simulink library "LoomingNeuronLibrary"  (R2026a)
settings: Solver=VariableStepAuto
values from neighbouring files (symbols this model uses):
  K_photoD = 1.1536    [FFIModelParams_16_02_2021.m]
  K_photoP = 6.8945    [FFIModelParams_16_02_2021.m]
undefined symbols (not defined in the file or in its folder): alpha_1, alpha_2, DiscIntNeverNeededParam, randi, retinaStencil, tau
libraries: simulink x4, $bdroot x2

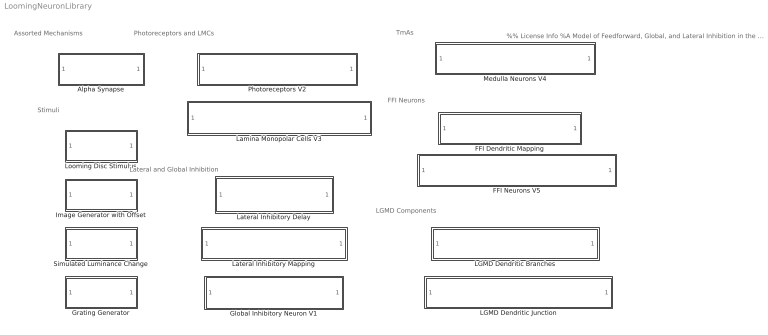
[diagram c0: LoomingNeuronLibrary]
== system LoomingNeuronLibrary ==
  note: TmAs
  note: FFI Neurons
  note: LGMD Components
  note: Lateral and Global Inhibition
  note: Photoreceptors and LMCs
  note: Stimuli
  note: Assorted Mechanisms
  note: %% License Info %A Model of Feedforward, Global, and Lateral Inhibition in the Locust Visual System. %This model examines the architecture and function of inhibitory mechanisms in the %visual system of locusts, namely those involved in the processing of inputs to a %key looming-sensitive neuron, the lobula giant movement detector (LGMD). %Copyright (c) 2026, Erik Olson, Travis Wiens, and Jack Gray %CITATION: %When using the model code for scientific publications, cite the following work: %Olson EGN, Wiens TK, Gray JR. A model of feedforward, global, and lateral inhibition %in the locust visual system predicts responses to looming stimuli. Biol Cybern. 2021 %Jun;115(3):245-265. doi: 10.1007/s00422-021-00876-8. Epub 2021 May 16. PMID: 33997912. %This program is free software: you can redistribute it and/or modify %it under the terms of the GNU General Public License as published by %the Free Software Foundation, either version 3 of the License, or %(at your option) any later version. %This program is distributed in the hope that it will be useful, %but WITHOUT ANY WARRANTY; without even the implied warranty of %MERCHANTABILITY or FITNESS FOR A PARTICULAR PURPOSE. See the %GNU General Public License for more details. %You should have received a copy of the GNU General Public License %along with this program. If not, see <https://www.gnu.org/licenses/>. %Contact: erik.olson@usask.ca
  Alpha Synapse : Subsystem  mask(Synaptic conductance function){tau=tau}
      mask prompts: tau "Synaptic time constant [s]"
      mask help: This block describes an alpha synapse with a single time constant, tau [s] governing peak time and decay. The output is normalized to a peak value of 1.
  FFI Dendritic Mapping : Subsystem  mask(FFI Neuron Dendrites){r_f=0, r_s=0, pop_FFI=0}
      mask prompts: r_f "Receptive field radius"; r_s "Receptive field spacing"; pop_FFI "FFI neuron population size"
      mask help: This block groups LMC outputs into receptive fields corresponding to each FFI neuron. These receptive fields are distributed in a manner mirroring the hexagonal arrangement of the retinotopic units, but with wider spacing of multiple retinotopic units (specified in the parameters). These receptive fields are similarly hexagonal, with sizes specified as a radius in retinotopic units. Inputs: Inputs: TmA Outputs = nondimensionalized alpha synapse outputs from TmAs. Outputs: Inputs to FFI Neurons = vector with elements corresponding to the population size of FFI neurons. Each value represents non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
  FFI Neurons V5 : Subsystem  mask(Feedforward Inhibitory Neurons){K_in=0, g_m=0, c_m=0.1, E_rev=0, E_rest=0, V_t=0, Delta_t=0.001, V_fire=0, tau=0.003, g_FFI_adap=0, tau_FFI_adap=0, E_adap=0, g_noise=0, noise_T=0, pop=0}
      mask prompts: K_in "Input conductance gain"; g_m "Membrane conductance [S/m^2]"; c_m "Membrane capacitance [F/m^2]"; E_rev "Input reversal potential [V]"; E_rest "Membrane resting potential [V]"; V_t "Sodium channel threshold [V]"; Delta_t "Spike initiation sharpness [V]"; V_fire "Firing voltage [V]"; tau "Synaptic decay constant [s]"; g_FFI_adap "Adaptation increment [S/m^2]"; tau_FFI_adap "Adaptation decay constant [s]"; E_adap "Adaptation reversal potential [V]"; g_noise "Noise amplitude [S/m^2]"; noise_T "Noise correlation time [s]"; pop "FFI neuron population size"
      mask help: Models a population of medullary neurons in the locust responsible for feedforward inhibition to the LGMD. Inputs from the lamina should be routed through the corresponding block "FFI Dendritic Mapping" before being supplied to this component. The neurons use an Exponential-Integrate-and-Fire (EIF) Model, incorporating an exponential activation function for sodium currents. The threshold voltage governing these channels is specified separately from the voltage used in spike determination. The neurons also incorporate adaptation currents, albeit without voltage coupling. Noise is also present i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
  Global Inhibitory Neuron V1 : Subsystem  mask(Nonspiking Global Inhibitory Neuron){K_in=0}
      mask prompts: K_in "Input gain [1/V]"
      mask help: This block represents a network of gap junction-connected, nonspiking neurons, receiving excitatory inputs from individual lamina units and generating an inhibitory signal applied across the medulla. The output approaches a limit asymptotically as the input strength increases, simulating the membrane voltage approaching the reversal potential of the input channels. Inputs: Summed LMC Activity = LMC membrane voltages, summed across the entire retina [V] Outputs: Global Inhibitory Signal = nondimensional signal ranging from 0 asymptotically toward a maximum possible value of 1, representing glob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
  Grating Generator : Subsystem  mask{radius=49, theta_max=pi, gratingPeriod=0.2}
      mask prompts: radius "Radius of the eye, in ommatidia"; theta_max "Maximum visual subtense of the eye [rad]"; gratingPeriod "Grating period [rad]"
      mask help: Generates a patch of sinusoidal black and white grating in the center of the visual field, which can move as the "position" input changes. The image background is white. Values regarding the size of the eye in terms of ommatidia and subtense angle are specified in the parameters field. "Grating period" describes the spacing between the dark stripes on the grating. Note that the grating region is rounded up in size to fully occupy any ommatidia near its edge. Inputs: theta = the visual subtense angle of the grating [radians] position = the angular position of the grating [rad]. Increasing or de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
  Image Generator with Offset : Subsystem  mask{radius=49, theta_max=pi, h_offset=0, v_offset=0}
      mask prompts: radius "Radius, in ommatidia"; theta_max "Maximum visual subtense [rad]"; h_offset "Axis 1 offset of image, in ommatidia"; v_offset "Axis 2 offset of image"
      mask help: Generates an array of luminance inputs to a simulated compound eye. These inputs correspond to the image of an approaching black disc-shaped object on a white background. The data is stored in a portion of a square array with the corners removed, corresponding to a hexagonal array of hexagonal ommatidia. The center of the image can be offset from the center of the eye along two axes by integer numbers of ommatidia. Due to the hexagonal nature of the ommatidial arrangement, these two axes are 60 degrees apart. Inputs: theta = the visual subtense angle of the object [radians] Outputs: image = a 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
  LGMD Dendritic Branches : Subsystem  mask(LGMD Dendritic Field A Branches){K_in=0, A_m=5e-6, G_m=0, G_b_j=0, C_m=1e-5, E_rev=0, E_rest=-0.07}
      mask prompts: K_in "Input conductance gain [S]"; A_m "Membrane area [m^2]"; G_m "Membrane conductance [S/m^2]"; G_b_j "Dendrite-soma conductance [S]"; C_m "Membrane capacitance [F/m^2]"; E_rev "Input reversal potential [V]"; E_rest "Resting potential [V]"
      mask help: A simulation of the branches of LGMD dendritic field A for a compartmental model. Inputs: TmA Outputs = nondimensionalized alpha synapse outputs from TmAs; these must first be correctly mapped into a vector corresponding in size to the number of dendritic branches. Dendritic Junction Membrane Voltage = membrane potential [V] of the attached dendritic junction compartment, used to determine intercompartmental currents. Outputs: Dendrite Voltages = vector of membrane potentials [V] of the modelled dendrites, used for monitoring purposes. Output Current = total output current from the dendrititic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
  LGMD Dendritic Junction : Subsystem  mask(LGMD Dendritic Field A Branches){A_m=5e-9, G_j_c=0, G_m=1.1, C_m=0.015, E_rest=0}
      mask prompts: A_m "Membrane Area [m^2]"; G_j_c "Junction-calcium conductance [S]"; G_m "Membrane conductance [S/m^2]"; C_m "Membrane capacitance [F/m^2]"; E_rest "Resting potential [mV]"
      mask help: A simulation of the proximal portion of LGMD dendritic field A. Inputs: Calcium Compartment Membrane Voltage = membrane potential [V] of the attached calcium compartment, used to determine intercompartmental currents. Dendritic Currents = total input current from the dendrititic branches to the dendritic junction compartment [A]. Outputs: Output Currents = total output current from the dendrititic junction to the calcium compartment [A]. Membrane Voltage = membrane potential [V] of the dendritic junction, used for monitoring purposes.
  Lamina Monopolar Cells V3 : Subsystem  mask(Locust Lamina Monopolar Cells){K_LMC=0, gamma_1=0}
      mask prompts: K_LMC "Gain [1/s]"; gamma_1 "Pole [1/s]"
      mask help: A representation of locust lamina monopolar cells. Uses a first-order transfer function with a single zero to approximate the response of lamina monopolar cell membrane voltage to photoreceptor membrane voltage. The response modelled is purely transient. Inputs: Photoreceptor Membrane Voltages = membrane potentials [V] of the photoreceptor corresponding to the modelled LMC, or an array thereof Outputs: LMC Membrane Voltages = membrane potentials [V] of corresponding dimensionality to the luminance inputs (either single or an array).
  Lateral Inhibitory Delay : Subsystem  mask(Lateral Inhibitory Delay){tau=1}
      mask prompts: tau "Time constant [s]"
      mask help: A first order low-pass filter, used to delay and temporally broaden LMC excitatory signals for use as lateral inhibition. LMC Activity = membrane potentials [V] of modelled LMCs, in array format Outputs: Lateral Inhibitory Signals = delayed and broadened LMC outputs [V], prior to mapping to adjacent retinotopic units.
  Lateral Inhibitory Mapping : Subsystem  mask(Lamina Output Mapping){stencil=0}
      mask prompts: stencil "Convolution kernel"
      mask help: This block maps signals from adjacent lamina cells to medullary neurons by using a supplied stencil to perform a 2D convolution. Inputs: Lamina Outputs = an array of LMC membrane potentials delayed via low-pass filter [V] Outputs: Lateral Inhibitory Signals = an array of inputs to the TmAs, corresponding to outputs of retinotopically adjacent LMCs, with radius and weightings determined by the kernel used for convolution
  Looming Disc Stimulus : Subsystem  mask(Looming Disc Stimulus){l=.07, v=3, d_0=0}
      mask prompts: l "stimulus half-height [m]"; v "stimulus approach velocity [m/s]"; d_0 "starting distance [m]"
      mask help: To be used in modelling visual parameters of a looming disc-shaped object, based on its half-height, approach velocity, and starting distance. Outputs include: theta = the visual subtense angle [rad] t_collision = simulation time normalized to the time of collision [s], such that negative values represent time pre-collision
  Medulla Neurons V4 : Subsystem  mask(Trans-medullary Afferents){K_in_ex=0, K_in_lateral=0, K_in_global=0, g_m=0, c_m=0.01, E_rev_ex=0, E_rev_inh=0, E_rest=0, V_t=0, Delta_t=0.001, V_fire=0, tau=0.0003, g_med_adap_inc=0, tau_med_adap=0.1, E_rev_adap=0, g_noise=0, noise_T=0.01, radius=1}
      mask prompts: K_in_ex "Excitatory conductance gain [S/(m^2*V)]"; K_in_lateral "Lateral inhibition conductance gain [S/(m^2*V)]"; K_in_global "Global inhibition conductance gain [S/(m^2)]"; g_m "Membrane conductance [S/m^2]"; c_m "Membrane capacitance [F/m^2]"; E_rev_ex "Excitatory reversal potential [V]"; E_rev_inh "Inhibitory reversal potential [V]"; E_rest "Membrane resting potential [V]"; V_t "Spike initiation threshold [V]"; Delta_t "Spike initiation sharpness [V]"; V_fire "Firing voltage [V]"; tau "Synaptic decay constant [s]"; g_med_adap_inc "Adaptation conductance increment [S/m^2]"; tau_med_adap "Adaptation time constant [s]"; E_rev_adap "Adaptation reversal potential [V]"; g_noise "Noise amplitude [S/m^2]"; noise_T "Noise correlation time [s]"; radius "Radius, in ommatidia"
      mask help: These neurons are meant to receive excitatory inputs from a retinotopically correspondent LMC, along with lateral inhibition based on adjacent LMC behaviour and global inhibition based on summed LMC behavior. They use an Exponential-Integrate-and-Fire (EIF) Model, incorporating an exponential activation function for spike initiation representing the function of voltage-gated sodium channels. The threshold voltage governing these channels is specified separately from the voltage used in spike determination. An adaptation current is also implemented; this does not include a voltage coupling term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
  Photoreceptors V2 : Subsystem  mask(Locust Photoreceptors){K_photoD=K_photoD, K_photoP=K_photoP, alpha_1=alpha_1, alpha_2=alpha_2}
      mask prompts: K_photoD "Derivative coefficient [V/s]"; K_photoP "Proportional coefficient [V/s^2]"; alpha_1 "First pole [1/s]"; alpha_2 "Second pole [1/s]"
      mask help: A representation of locust photoreceptors. Uses a 2nd-order transfer function with a single zero to model the response of membrane voltage to luminance, incorporating a transient overshoot and a steady-state component. Inputs: Luminance Values = either a single luminance value ranging from 1 (white) to 0 (black) representing visual input from the corresponding ommatidium, or an array thereof,. Outputs: Photoreceptor Membrane Voltages = membrane voltage of photoreceptors [V], of corresponding dimensionality to the luminance inputs (either single or an array).
  Simulated Luminance Change : Subsystem  mask(Simulated Luminance Change){duration=1, start=0}
      mask prompts: duration "Duration [s]"; start "Start time [s]"
      mask help: Simulates the luminance change from dark to light to over a single ommatidium due to an edge moving at constant speed. Used to implement single-facet stimuli . The luminance corresponds to the potion of a circular region covered by a straight line passing across it at constant speed. Outputs: luminance = a luminance value transition from 1 (white) to 0 (black), starting at the specified time and ending after the specified duration.

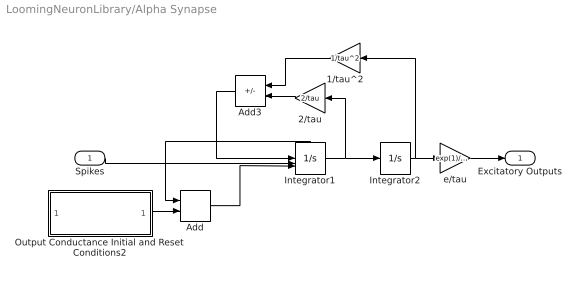
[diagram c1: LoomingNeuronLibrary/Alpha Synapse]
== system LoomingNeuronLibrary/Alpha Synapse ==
  Spikes : Inport
  1/tau^2 : Gain  Gain=1/tau^2
  2/tau : Gain  Gain=2/tau
  Add : Sum
  Add3 : Sum  Inputs=--
  Integrator1 : Integrator  ExternalReset=rising  InitialConditionSource=external  ShowStatePort=on
  Integrator2 : Integrator
  Output Conductance Initial and Reset Conditions2 : Subsystem
  e/tau : Gain  Gain=exp(1)/tau
  Excitatory Outputs : Outport  VectorParamsAs1DForOutWhenUnconnected=off
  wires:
  Add3/1 -> Integrator1/1
  Integrator2/1 -> 1/tau^2/1, e/tau/1
  e/tau/1 -> Excitatory Outputs/1
  Output Conductance Initial and Reset Conditions2/1(Reset Value) -> Add/2
  1/tau^2/1 -> Add3/1
  Add/1 -> Integrator1/3
  Integrator1/1 -> 2/tau/1, Integrator2/1
  Integrator1/State -> Add/1
  Spikes/1 -> Integrator1/2
  2/tau/1 -> Add3/2

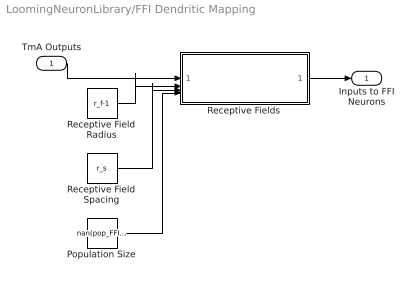
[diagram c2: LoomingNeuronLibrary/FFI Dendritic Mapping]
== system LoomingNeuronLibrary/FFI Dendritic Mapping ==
  TmA Outputs : Inport
  Population Size : Constant  Value=nan(pop_FFI,1)
  Receptive Field Radius : Constant  Value=r_f-1
  Receptive Field Spacing : Constant  Value=r_s
  Receptive Fields : MATLAB Function  TreatAsAtomicUnit=on
  Inputs to FFI Neurons : Outport  VectorParamsAs1DForOutWhenUnconnected=off
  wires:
  Population Size/1 -> Receptive Fields/4(output_array)
  Receptive Field Spacing/1 -> Receptive Fields/3(r_s)
  TmA Outputs/1 -> Receptive Fields/1(LMCs)
  Receptive Field Radius/1 -> Receptive Fields/2(r_f)
  Receptive Fields/1(y) -> Inputs to FFI Neurons/1

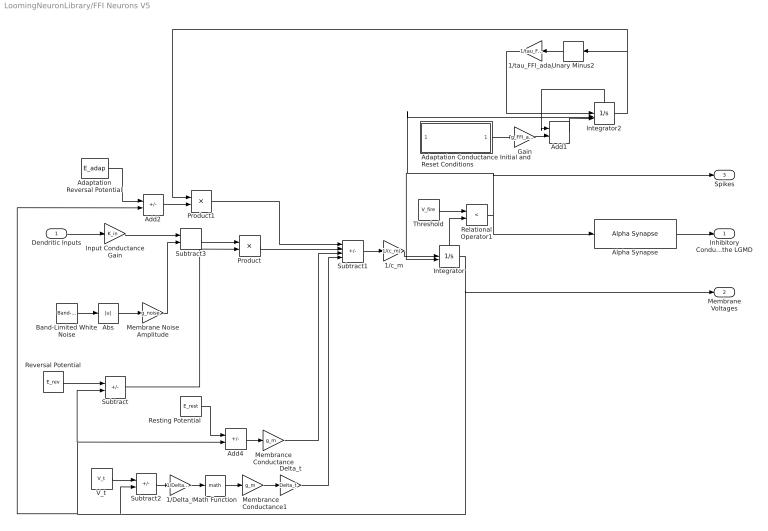
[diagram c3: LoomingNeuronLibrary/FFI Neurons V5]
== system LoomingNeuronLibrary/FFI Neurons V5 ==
  Dendritic Inputs : Inport
  1/Delta_t : Gain  Gain=1/Delta_t
  1/c_m : Gain  Gain=1/(c_m)
  1/tau_FFI_adap : Gain  Gain=1/tau_FFI_adap
  Abs : Abs
  Adaptation Reversal Potential : Constant  Value=E_adap
  Adaptation Conductance Initial and Reset Conditions : Subsystem
  Add1 : Sum
  Add2 : Sum  Inputs=-+
  Add4 : Sum  Inputs=-+
  Alpha Synapse : $bdroot/Alpha Synapse  tau=tau
  Band-Limited White Noise : simulink/Sources/Band-Limited White Noise  Cov=[noise_T]  Ts=noise_T  seed=randi(1000000,pop,1)
  Delta_t : Gain  Gain=Delta_t
  Gain : Gain  Gain=g_FFI_adap
  Input Conductance Gain : Gain  Gain=K_in
  Integrator : Integrator  ExternalReset=rising  InitialCondition=E_rest  ShowStatePort=on
  Integrator2 : Integrator  ExternalReset=rising  InitialConditionSource=external  ShowStatePort=on
  Math Function : Math  SignedPower=on
  Membrance Conductance : Gain  Gain=g_m
  Membrance Conductance1 : Gain  Gain=g_m
  Membrane Noise Amplitude : Gain  Gain=g_noise
  Product : Product
  Product1 : Product
  Relational Operator1 : RelationalOperator  Operator=<  OutDataTypeStr=boolean  RndMeth=Simplest
  Resting Potential : Constant  Value=E_rest
  Reversal Potential : Constant  Value=E_rev
  Subtract : Sum  Inputs=+-
  Subtract1 : Sum  Inputs=-+-+
  Subtract2 : Sum  Inputs=-+
  Subtract3 : Sum
  Threshold : Constant  Value=V_fire
  Unary Minus2 : UnaryMinus
  V_t : Constant  Value=V_t
  Inhibitory Conductance Outputs to the LGMD : Outport  VectorParamsAs1DForOutWhenUnconnected=off
  Membrane Voltages : Outport  Port=2  VectorParamsAs1DForOutWhenUnconnected=off
  Spikes : Outport  Port=3  VectorParamsAs1DForOutWhenUnconnected=off
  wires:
  Threshold/1 -> Relational Operator1/1
  Subtract/1 -> Product/2
  Subtract1/1 -> 1/c_m/1
  Resting Potential/1 -> Add4/1
  Dendritic Inputs/1 -> Input Conductance Gain/1
  1/c_m/1 -> Integrator/1
  Integrator/State -> Relational Operator1/2
  Reversal Potential/1 -> Subtract/1
  Add4/1 -> Membrance Conductance/1
  Subtract2/1 -> 1/Delta_t/1
  Delta_t/1 -> Subtract1/4
  Math Function/1 -> Membrance Conductance1/1
  1/Delta_t/1 -> Math Function/1
  Membrance Conductance1/1 -> Delta_t/1
  V_t/1 -> Subtract2/1
  1/tau_FFI_adap/1 -> Integrator2/1
  Integrator2/State -> Add1/1
  Unary Minus2/1 -> 1/tau_FFI_adap/1
  Relational Operator1/1 -> Alpha Synapse/1, Spikes/1, Integrator2/2, Integrator/2
  Add1/1 -> Integrator2/3
  Gain/1 -> Add1/2
  Integrator2/1 -> Unary Minus2/1, Product1/1
  Product1/1 -> Subtract1/1
  Add2/1 -> Product1/2
  Integrator/1 -> Membrane Voltages/1, Subtract2/2, Add4/2, Subtract/2, Add2/2
  Adaptation Reversal Potential/1 -> Add2/1
  Membrance Conductance/1 -> Subtract1/3
  Product/1 -> Subtract1/2
  Band-Limited White Noise/1 -> Abs/1
  Membrane Noise Amplitude/1 -> Subtract3/2
  Abs/1 -> Membrane Noise Amplitude/1
  Subtract3/1 -> Product/1
  Input Conductance Gain/1 -> Subtract3/1
  Adaptation Conductance Initial and Reset Conditions/1(Reset Value) -> Gain/1
  Alpha Synapse/1 -> Inhibitory Conductance Outputs to the LGMD/1

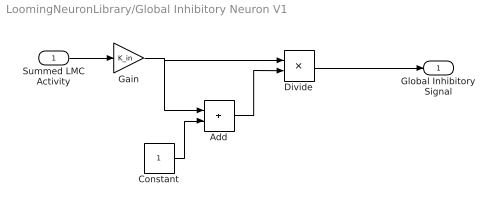
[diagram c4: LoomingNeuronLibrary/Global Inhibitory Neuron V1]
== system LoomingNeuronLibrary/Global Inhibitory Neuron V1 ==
  Summed LMC Activity : Inport
  Add : Sum
  Constant : Constant
  Divide : Product  Inputs=*/
  Gain : Gain  Gain=K_in
  Global Inhibitory Signal : Outport  VectorParamsAs1DForOutWhenUnconnected=off
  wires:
  Divide/1 -> Global Inhibitory Signal/1
  Summed LMC Activity/1 -> Gain/1
  Gain/1 -> Add/1, Divide/1
  Constant/1 -> Add/2
  Add/1 -> Divide/2

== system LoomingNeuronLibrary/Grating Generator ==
  theta : Inport
  position : Inport  Port=2
  Constant : Constant  Value=ones(2*radius-1, 2*radius-1)
  Constant1 : Constant  Value=gratingPeriod
  MATLAB Function : MATLAB Function  TreatAsAtomicUnit=on
  image : Outport  PortDimensions=[2*radius-1 2*radius-1]  VectorParamsAs1DForOutWhenUnconnected=off
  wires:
  theta/1 -> MATLAB Function/1(theta)
  MATLAB Function/1(image) -> image/1
  Constant/1 -> MATLAB Function/4(blank)
  position/1 -> MATLAB Function/2(position)
  Constant1/1 -> MATLAB Function/3(gratingPeriod)

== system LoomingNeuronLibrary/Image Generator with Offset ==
  theta : Inport
  Constant : Constant  Value=ones(2*radius-1, 2*radius-1)
  Constant1 : Constant  Value=h_offset
  Constant2 : Constant  Value=v_offset
  MATLAB Function : MATLAB Function  TreatAsAtomicUnit=on
  image : Outport  PortDimensions=[2*radius-1 2*radius-1]  VectorParamsAs1DForOutWhenUnconnected=off
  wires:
  theta/1 -> MATLAB Function/1(theta)
  MATLAB Function/1(image) -> image/1
  Constant/1 -> MATLAB Function/2(blank)
  Constant1/1 -> MATLAB Function/3(h_offset)
  Constant2/1 -> MATLAB Function/4(v_offset)

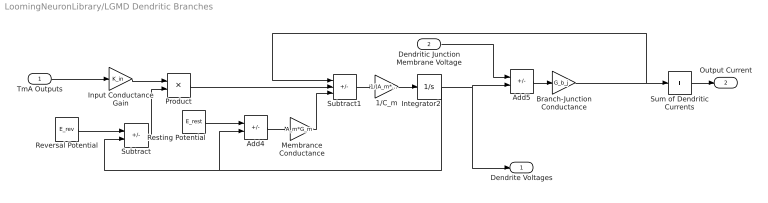
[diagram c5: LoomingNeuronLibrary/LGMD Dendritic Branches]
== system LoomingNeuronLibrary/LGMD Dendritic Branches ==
  TmA Outputs : Inport
  Dendritic Junction Membrane Voltage : Inport  Port=2
  1/C_m : Gain  Gain=1/(A_m*C_m)
  Add4 : Sum  Inputs=-+
  Add5 : Sum  Inputs=-+
  Branch-Junction Conductance : Gain  Gain=G_b_j
  Input Conductance Gain : Gain  Gain=K_in
  Integrator2 : Integrator  InitialCondition=E_rest
  Membrance Conductance : Gain  Gain=A_m*G_m
  Product : Product
  Resting Potential : Constant  Value=E_rest
  Reversal Potential : Constant  Value=E_rev
  Subtract : Sum  Inputs=+-
  Subtract1 : Sum  Inputs=-+-
  Sum of Dendritic Currents : Sum  Inputs=+
  Dendrite Voltages : Outport  VectorParamsAs1DForOutWhenUnconnected=off
  Output Current : Outport  Port=2  VectorParamsAs1DForOutWhenUnconnected=off
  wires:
  1/C_m/1 -> Integrator2/1
  Sum of Dendritic Currents/1 -> Output Current/1
  Integrator2/1 -> Add4/2, Subtract/2, Dendrite Voltages/1, Add5/2
  Subtract/1 -> Product/2
  Reversal Potential/1 -> Subtract/1
  Add4/1 -> Membrance Conductance/1
  Input Conductance Gain/1 -> Product/1
  Subtract1/1 -> 1/C_m/1
  Resting Potential/1 -> Add4/1
  TmA Outputs/1 -> Input Conductance Gain/1
  Dendritic Junction Membrane Voltage/1 -> Add5/1
  Product/1 -> Subtract1/2
  Membrance Conductance/1 -> Subtract1/3
  Add5/1 -> Branch-Junction Conductance/1
  Branch-Junction Conductance/1 -> Subtract1/1, Sum of Dendritic Currents/1

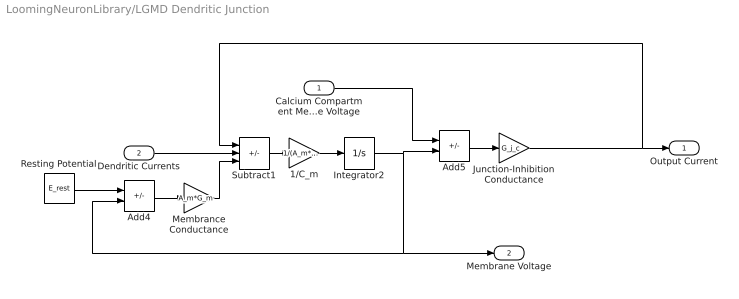
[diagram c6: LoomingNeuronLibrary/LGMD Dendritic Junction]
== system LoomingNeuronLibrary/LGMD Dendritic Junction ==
  Calcium Compartment Membrane Voltage : Inport
  Dendritic Currents : Inport  Port=2
  1/C_m : Gain  Gain=1/(A_m*C_m)
  Add4 : Sum  Inputs=-+
  Add5 : Sum  Inputs=-+
  Integrator2 : Integrator  InitialCondition=E_rest
  Junction-Inhibition Conductance : Gain  Gain=G_j_c
  Membrance Conductance : Gain  Gain=A_m*G_m
  Resting Potential : Constant  Value=E_rest
  Subtract1 : Sum  Inputs=-+-
  Output Current : Outport  VectorParamsAs1DForOutWhenUnconnected=off
  Membrane Voltage : Outport  Port=2  VectorParamsAs1DForOutWhenUnconnected=off
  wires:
  Membrance Conductance/1 -> Subtract1/3
  Add4/1 -> Membrance Conductance/1
  1/C_m/1 -> Integrator2/1
  Dendritic Currents/1 -> Subtract1/2
  Subtract1/1 -> 1/C_m/1
  Resting Potential/1 -> Add4/1
  Add5/1 -> Junction-Inhibition Conductance/1
  Calcium Compartment Membrane Voltage/1 -> Add5/1
  Junction-Inhibition Conductance/1 -> Output Current/1, Subtract1/1
  Integrator2/1 -> Add5/2, Membrane Voltage/1, Add4/2

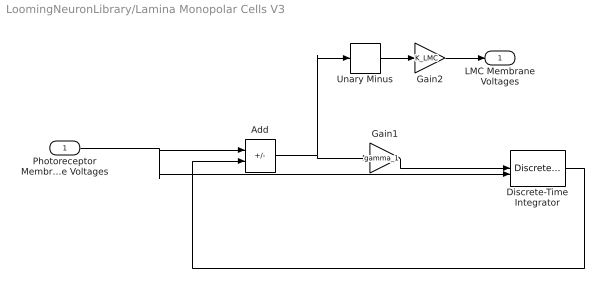
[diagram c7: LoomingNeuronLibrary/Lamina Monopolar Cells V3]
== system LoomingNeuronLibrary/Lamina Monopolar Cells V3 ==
  Photoreceptor Membrane Voltages : Inport
  Add : Sum  Inputs=+-
  Discrete-Time Integrator : DiscreteIntegrator  InitialConditionSource=external  SampleTime=-1  ICPrevOutput=DiscIntNeverNeededParam  ICPrevScaledInput=DiscIntNeverNeededParam
  Gain1 : Gain  Gain=gamma_1
  Gain2 : Gain  Gain=K_LMC
  Unary Minus : UnaryMinus
  LMC Membrane Voltages : Outport  VectorParamsAs1DForOutWhenUnconnected=off
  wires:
  Gain1/1 -> Discrete-Time Integrator/1
  Discrete-Time Integrator/1 -> Add/2
  Photoreceptor Membrane Voltages/1 -> Discrete-Time Integrator/2, Add/1
  Add/1 -> Unary Minus/1, Gain1/1
  Unary Minus/1 -> Gain2/1
  Gain2/1 -> LMC Membrane Voltages/1

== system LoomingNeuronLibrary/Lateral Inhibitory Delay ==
  LMC Activity : Inport
  Add : Sum  Inputs=+-
  Discrete-Time Integrator : DiscreteIntegrator  SampleTime=-1  ICPrevOutput=DiscIntNeverNeededParam  ICPrevScaledInput=DiscIntNeverNeededParam
  Gain : Gain  Gain=1/tau
  Lateral Inhibitory Signals : Outport
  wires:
  Discrete-Time Integrator/1 -> Lateral Inhibitory Signals/1, Add/2
  Add/1 -> Gain/1
  LMC Activity/1 -> Add/1
  Gain/1 -> Discrete-Time Integrator/1

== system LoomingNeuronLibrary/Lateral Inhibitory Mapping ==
  Lamina Outputs : Inport
  Constant : Constant  Value=stencil
  MATLAB Function : MATLAB Function  TreatAsAtomicUnit=on
  Lateral Inhibitory Signals : Outport  VectorParamsAs1DForOutWhenUnconnected=off
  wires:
  Lamina Outputs/1 -> MATLAB Function/1(LMCs)
  MATLAB Function/1(inhibition) -> Lateral Inhibitory Signals/1
  Constant/1 -> MATLAB Function/2(stencil)

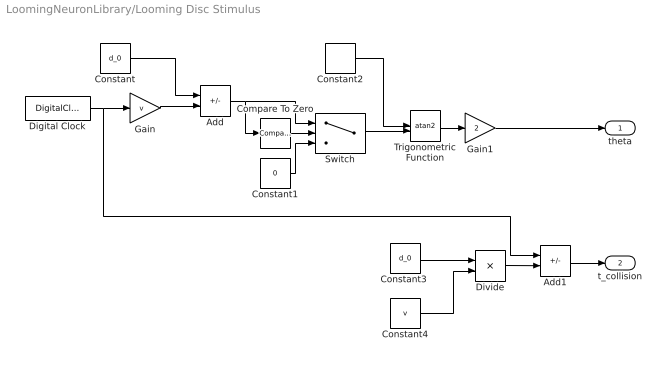
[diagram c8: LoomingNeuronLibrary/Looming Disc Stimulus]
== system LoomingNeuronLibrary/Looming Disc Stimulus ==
  Add : Sum  Inputs=+-
  Add1 : Sum  Inputs=+-
  Compare To Zero : simulink/Logic and Bit Operations/Compare To Zero  relop=>=  OutDataTypeStr=boolean
  Constant : Constant  Value=d_0
  Constant1 : Constant  Value=0
  Constant2 : Constant  Value=l
  "Constant3 " : Constant  Value=d_0
  Constant4 : Constant  Value=v
  Digital Clock : DigitalClock  SampleTime=-1
  Divide : Product  Inputs=*/
  Gain : Gain  Gain=v
  Gain1 : Gain  Gain=2
  Switch : Switch  Criteria=u2 > Threshold
  Trigonometric Function : Trigonometry  Operator=atan2  OutputSignalType=real
  theta : Outport  VectorParamsAs1DForOutWhenUnconnected=off
  t_collision : Outport  Port=2  VectorParamsAs1DForOutWhenUnconnected=off
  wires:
  Constant/1 -> Add/1
  Gain/1 -> Add/2
  Compare To Zero/1 -> Switch/2
  Digital Clock/1 -> Add1/1, Gain/1
  Add/1 -> Compare To Zero/1, Switch/1
  Constant1/1 -> Switch/3
  Trigonometric Function/1 -> Gain1/1
  Switch/1 -> Trigonometric Function/2
  Constant2/1 -> Trigonometric Function/1
  Gain1/1 -> theta/1
  "Constant3 "/1 -> Divide/1
  Constant4/1 -> Divide/2
  Divide/1 -> Add1/2
  Add1/1 -> t_collision/1

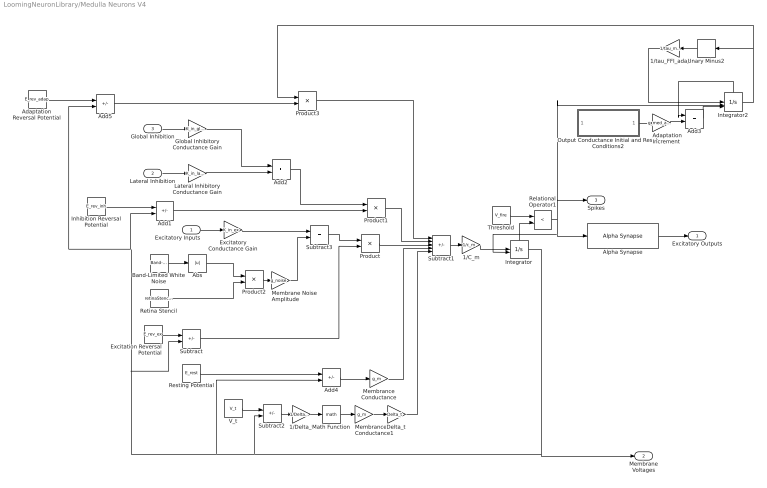
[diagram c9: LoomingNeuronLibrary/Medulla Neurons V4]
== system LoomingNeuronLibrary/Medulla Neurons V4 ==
  Excitatory Inputs : Inport
  Lateral Inhibition : Inport  Port=2
  Global Inhibition : Inport  Port=3
  1/C_m : Gain  Gain=1/c_m
  1/Delta_t : Gain  Gain=1/Delta_t
  1/tau_FFI_adap : Gain  Gain=1/tau_med_adap
  Abs : Abs
  Adaptation Increment : Gain  Gain=g_med_adap_inc
  Adaptation Reversal Potential : Constant  Value=E_rev_adap
  Add1 : Sum  Inputs=-+
  Add2 : Sum
  Add3 : Sum
  Add4 : Sum  Inputs=-+
  Add5 : Sum  Inputs=-+
  Alpha Synapse : $bdroot/Alpha Synapse  tau=tau
  Band-Limited White Noise : simulink/Sources/Band-Limited White Noise  Cov=[noise_T]  Ts=noise_T  seed=randi(1000000,2*radius-1)
  Delta_t : Gain  Gain=Delta_t
  Excitation Reversal Potential : Constant  Value=E_rev_ex
  Excitatory Conductance Gain : Gain  Gain=K_in_ex
  Global Inhibitory Conductance Gain : Gain  Gain=K_in_global
  Inhibition Reversal Potential : Constant  Value=E_rev_inh
  Integrator : Integrator  ExternalReset=rising  InitialCondition=E_rest  ShowStatePort=on
  Integrator2 : Integrator  ExternalReset=rising  InitialConditionSource=external  ShowStatePort=on
  Lateral Inhibitory Conductance Gain : Gain  Gain=K_in_lateral
  Math Function : Math  SignedPower=on
  Membrance Conductance : Gain  Gain=g_m
  Membrance Conductance1 : Gain  Gain=g_m
  Membrane Noise Amplitude : Gain  Gain=g_noise
  Output Conductance Initial and Reset Conditions2 : Subsystem
  Product{,1..3} (4 alike) : Product
  Relational Operator1 : RelationalOperator  Operator=<  OutDataTypeStr=boolean  RndMeth=Simplest
  Resting Potential : Constant  Value=E_rest
  Retina Stencil : Constant  Value=retinaStencil(radius)
  Subtract : Sum  Inputs=+-
  Subtract1 : Sum  Inputs=--+-+
  Subtract2 : Sum  Inputs=-+
  Subtract3 : Sum
  Threshold : Constant  Value=V_fire
  Unary Minus2 : UnaryMinus
  V_t : Constant  Value=V_t
  Excitatory Outputs : Outport  VectorParamsAs1DForOutWhenUnconnected=off
  Membrane Voltages : Outport  Port=2  VectorParamsAs1DForOutWhenUnconnected=off
  Spikes : Outport  Port=3  VectorParamsAs1DForOutWhenUnconnected=off
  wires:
  Global Inhibition/1 -> Global Inhibitory Conductance Gain/1
  Integrator/State -> Relational Operator1/2
  Product/1 -> Subtract1/3
  Excitation Reversal Potential/1 -> Subtract/1
  Resting Potential/1 -> Add4/1
  Product1/1 -> Subtract1/2
  Delta_t/1 -> Subtract1/5
  1/Delta_t/1 -> Math Function/1
  Threshold/1 -> Relational Operator1/1
  Add4/1 -> Membrance Conductance/1
  Subtract2/1 -> 1/Delta_t/1
  Math Function/1 -> Membrance Conductance1/1
  Subtract/1 -> Product/2
  V_t/1 -> Subtract2/1
  Membrance Conductance/1 -> Subtract1/4
  Excitatory Inputs/1 -> Excitatory Conductance Gain/1
  Alpha Synapse/1 -> Excitatory Outputs/1
  Membrance Conductance1/1 -> Delta_t/1
  Subtract1/1 -> 1/C_m/1
  Lateral Inhibition/1 -> Lateral Inhibitory Conductance Gain/1
  Inhibition Reversal Potential/1 -> Add1/1
  1/C_m/1 -> Integrator/1
  Add2/1 -> Product1/1
  Add1/1 -> Product1/2
  Lateral Inhibitory Conductance Gain/1 -> Add2/2
  Global Inhibitory Conductance Gain/1 -> Add2/1
  Relational Operator1/1 -> Integrator2/2, Spikes/1, Integrator/2, Alpha Synapse/1
  1/tau_FFI_adap/1 -> Integrator2/1
  Integrator2/State -> Add3/1
  Add3/1 -> Integrator2/3
  Adaptation Increment/1 -> Add3/2
  Unary Minus2/1 -> 1/tau_FFI_adap/1
  Integrator2/1 -> Unary Minus2/1, Product3/1
  Excitatory Conductance Gain/1 -> Subtract3/1
  Subtract3/1 -> Product/1
  Membrane Noise Amplitude/1 -> Subtract3/2
  Product2/1 -> Membrane Noise Amplitude/1
  Band-Limited White Noise/1 -> Abs/1
  Retina Stencil/1 -> Product2/2
  Abs/1 -> Product2/1
  Output Conductance Initial and Reset Conditions2/1(Reset Value) -> Adaptation Increment/1
  Adaptation Reversal Potential/1 -> Add5/1
  Integrator/1 -> Subtract2/2, Add4/2, Add5/2, Add1/2, Subtract/2, Membrane Voltages/1
  Add5/1 -> Product3/2
  Product3/1 -> Subtract1/1

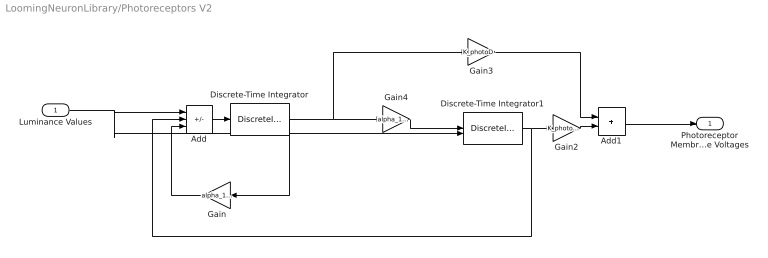
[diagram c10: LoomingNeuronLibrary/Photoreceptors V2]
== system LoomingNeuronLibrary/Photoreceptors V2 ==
  Luminance Values : Inport
  Add : Sum  Inputs=+--
  Add1 : Sum
  Discrete-Time Integrator : DiscreteIntegrator  SampleTime=-1  ICPrevOutput=DiscIntNeverNeededParam  ICPrevScaledInput=DiscIntNeverNeededParam
  Discrete-Time Integrator1 : DiscreteIntegrator  InitialConditionSource=external  SampleTime=-1  ICPrevOutput=DiscIntNeverNeededParam  ICPrevScaledInput=DiscIntNeverNeededParam
  Gain : Gain  Gain=alpha_1+alpha_2
  Gain2 : Gain  Gain=K_photoP/(alpha_1*alpha_2)
  Gain3 : Gain  Gain=K_photoD
  Gain4 : Gain  Gain=alpha_1*alpha_2
  Photoreceptor Membrane Voltages : Outport  VectorParamsAs1DForOutWhenUnconnected=off
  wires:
  Gain4/1 -> Discrete-Time Integrator1/1
  Luminance Values/1 -> Discrete-Time Integrator1/2, Add/1
  Add/1 -> Discrete-Time Integrator/1
  Discrete-Time Integrator1/1 -> Add/2, Gain2/1
  Gain/1 -> Add/3
  Gain2/1 -> Add1/2
  Gain3/1 -> Add1/1
  Add1/1 -> Photoreceptor Membrane Voltages/1
  Discrete-Time Integrator/1 -> Gain/1, Gain4/1, Gain3/1

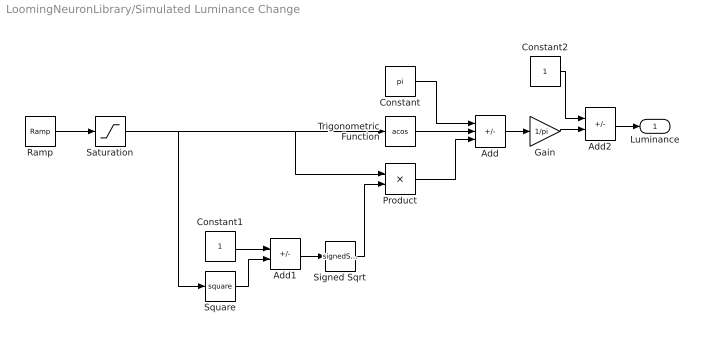
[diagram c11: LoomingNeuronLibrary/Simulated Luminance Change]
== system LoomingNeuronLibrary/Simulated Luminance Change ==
  Add : Sum  Inputs=+-+
  Add1 : Sum  Inputs=+-
  Add2 : Sum  Inputs=+-
  Constant : Constant  Value=pi
  Constant1 : Constant
  Constant2 : Constant
  Gain : Gain  Gain=1/pi
  Product : Product
  Ramp : simulink/Sources/Ramp  slope=2/duration  start=start  InitialOutput=-1
  Saturation : Saturate  UpperLimit=1  LowerLimit=-1
  Signed Sqrt : Sqrt  Operator=signedSqrt
  Square : Math  Operator=square  SignedPower=on
  Trigonometric Function : Trigonometry  Operator=acos
  Luminance : Outport  VectorParamsAs1DForOutWhenUnconnected=off
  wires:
  Saturation/1 -> Square/1, Trigonometric Function/1, Product/1
  Trigonometric Function/1 -> Add/2
  Product/1 -> Add/3
  Square/1 -> Add1/2
  Constant1/1 -> Add1/1
  Signed Sqrt/1 -> Product/2
  Add/1 -> Gain/1
  Ramp/1 -> Saturation/1
  Add1/1 -> Signed Sqrt/1
  Constant/1 -> Add/1
  Gain/1 -> Add2/2
  Constant2/1 -> Add2/1
  Add2/1 -> Luminance/1

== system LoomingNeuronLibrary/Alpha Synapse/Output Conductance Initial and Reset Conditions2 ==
  Clock : Clock
  Constant4 : Constant
  Constant5 : Constant  Value=0
  Switch1 : Switch  Criteria=u2 > Threshold
  Reset Value : Outport  VectorParamsAs1DForOutWhenUnconnected=off
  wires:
  Constant5/1 -> Switch1/3
  Switch1/1 -> Reset Value/1
  Constant4/1 -> Switch1/1
  Clock/1 -> Switch1/2

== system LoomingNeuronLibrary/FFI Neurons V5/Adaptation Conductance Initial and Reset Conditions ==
  Clock : Clock
  Constant4 : Constant
  Constant5 : Constant  Value=0
  Switch1 : Switch  Criteria=u2 > Threshold
  Reset Value : Outport  VectorParamsAs1DForOutWhenUnconnected=off
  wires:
  Clock/1 -> Switch1/2
  Constant4/1 -> Switch1/1
  Switch1/1 -> Reset Value/1
  Constant5/1 -> Switch1/3

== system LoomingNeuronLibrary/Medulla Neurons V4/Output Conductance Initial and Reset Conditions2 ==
  Clock : Clock
  Constant4 : Constant
  Constant5 : Constant  Value=0
  Switch1 : Switch  Criteria=u2 > Threshold
  Reset Value : Outport  VectorParamsAs1DForOutWhenUnconnected=off
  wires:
  Constant5/1 -> Switch1/3
  Switch1/1 -> Reset Value/1
  Constant4/1 -> Switch1/1
  Clock/1 -> Switch1/2

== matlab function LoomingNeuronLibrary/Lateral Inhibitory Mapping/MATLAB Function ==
function inhibition = lateralInhibition(LMCs,stencil)
inhibition = conv2(LMCs,stencil,'same');

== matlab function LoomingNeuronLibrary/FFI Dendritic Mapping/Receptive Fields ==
function y = fcn(LMCs,r_f,r_s,output_array)
%r_f in the radius of the receptive field in retinotopic units.  The center
%unit IS NOT counted.

diameter = size(LMCs,1);%width of the retina
radius = (diameter-1)/2+1;%number of retinotopic units (or ommatidia) counted 
                        %in either direction from the center of the retina.
                        %The center unit IS counted.
retina_bounds = ones(diameter)-triu(ones(diameter),radius)-tril(ones(diameter),-radius);

radius_f = floor(((diameter-1)/2)/r_s);%number of receptive fields, counted 
                                    %in either direction from the center of
                                    %the retina.  The center field IS NOT
                                    %counted.

receptive_convolution = ones(2*r_f+1)-triu(ones(2*r_f+1),r_f+1)-tril(ones(2*r_f+1),-1*(r_f+1));

padded_input = zeros(2*r_f+diameter);
padded_input(r_f+1:diameter+r_f,r_f+1:diameter+r_f) = LMCs.*retina_bounds;

count = 1;

for i = -radius_f:radius_f
    for j = -radius_f:radius_f
        if abs(i-j)<(radius_f+1)%check if this unit is within the hexagonal pattern
            center_horz = r_f+radius+i*r_s;
            center_vert = r_f+radius+j*r_s;
            output_array(count) = sum(padded_input(center_horz-r_f:center_horz+r_f,center_vert-r_f:center_vert+r_f).*receptive_convolution,'all');
            count = count+1;
        end
    end
end

y = output_array;

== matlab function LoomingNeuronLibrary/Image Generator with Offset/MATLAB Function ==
function image = offsetLuminanceImage(theta,theta_max,blank,h_offset,v_offset)
%this function generates a hexagonal array of hexagonal pixels with 
%different luminance values representing a 90 deg widevisual field image of 
%a dark looming object on a white background.  The data is stored in an array
%with the corners ignored (i.e. a hexagon) Inputs:
%theta = the visual subtense angle of the object [rad]
%theta_max = the maximum visual subtense angle of the image [rad]
%radius = the number of pixels from the center of the image to the edge,
%including the center.

omRadius = (size(blank,1)+1)/2;
image = blank;%create an array of appropriate size to 
%store the image
edgeRad = theta/theta_max*(omRadius-0.5);%distance from the edge of the object to 
%the center of the image, measured in hexagonal cell widths
lum = NaN(1,omRadius);%stores luminance values at different distances from 
%the center of the image.  The array index corresponds to the number of 
%cells away from the image center, starting at 1 for the center cell.
%a value of 0 corresponds to 100% black (covered by the object, 1 to 100% 
%white (uncovered by the object).  The cells are approximated as circular
relPos = edgeRad;%position of the object edge relative to the current cell

if relPos >= 0.5%if object edge is beyond the current cell
    lum(1) = 0;%set luminance to black
else
    lum(1) = 1-(2*relPos)^2;%set luminance to percentage of cell not 
    %covered
end
for i = 2:omRadius
    relPos = edgeRad-i+1;%position of the object edge relative to the 
    %current cell
    if relPos <= -0.5%if object is not yet at the current cell
        lum(i) = 1;%set luminance to white
    elseif relPos >= 0.5%if object edge is beyond the current cell
        lum(i) = 0;%set luminance to black
    else
        lum(i) = (acos(2*relPos)-2*relPos*sqrt(1-(2*relPos)^2))/pi;%set 
        %luminance to percentage of cell not covered
    end
end

for i = 1:2*omRadius-1%iterate through each element of the image
    for j = 1:2*omRadius-1
        if and(i-j < omRadius,i-j > -1*omRadius)%check if element is part of 
            %image
            rho = max([abs(i-omRadius),abs(j-omRadius),abs(i-j)])+1;%find distance from center of image
            image(i,j) = lum(rho);%set luminance value appropriately            
        else
            image(i,j) = 1;%if not, set to one
        end
    end
end

image_temp = blank;
image_temp(1+h_offset:end,1+h_offset+v_offset:end) = image(1:end-h_offset,1:end-h_offset-v_offset);
image = image_temp;

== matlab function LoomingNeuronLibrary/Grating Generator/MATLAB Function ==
function image = symmetricLuminanceImageV2(theta,position,gratingPeriod,theta_max,blank)

omRadius = (size(blank,1)+1)/2;
image = ones(size(blank));%create an array of appropriate size to 
%store the image
gridWidth = 2*ceil(theta/theta_max*(omRadius-0.5)+0.5)-1;%width of the grid
gratingPos1 = linspace(0,gridWidth-1,gridWidth)-floor(gridWidth/2);

angularSeparation = theta_max/size(blank,1);%*(sqrt(3)/2) the angular separation
%of the rows of the grating in radians
gratingPos1 = gratingPos1*angularSeparation;%angular positions of the grating rows
gratingPos1 = gratingPos1+position;%angular positions accounting for grating motion
gratingPos1 = 2*pi*gratingPos1/gratingPeriod;%angular positions in radians, 
%normalized to the grid stripe spacing
gratingPos2 = gratingPos1+gratingPos1(2)-gratingPos1(1);%angular positions offset by one row

gratingValues = ((sin(gratingPos2)-sin(gratingPos1))+(gratingPos2-gratingPos1))/(2*(gratingPos2(1)-gratingPos1(1)));

grating = ones(gridWidth,1)*gratingValues;

gratingStencil = tril(ones(gridWidth),ceil(gridWidth/2)-1)-tril(ones(gridWidth),-ceil(gridWidth/2));

grating = grating.*gratingStencil+ones(gridWidth,gridWidth)-gratingStencil;

gratingPosition = omRadius-ceil(gridWidth/2);

image(gratingPosition+1:gratingPosition+gridWidth,gratingPosition+1:gratingPosition+gridWidth) = grating;
